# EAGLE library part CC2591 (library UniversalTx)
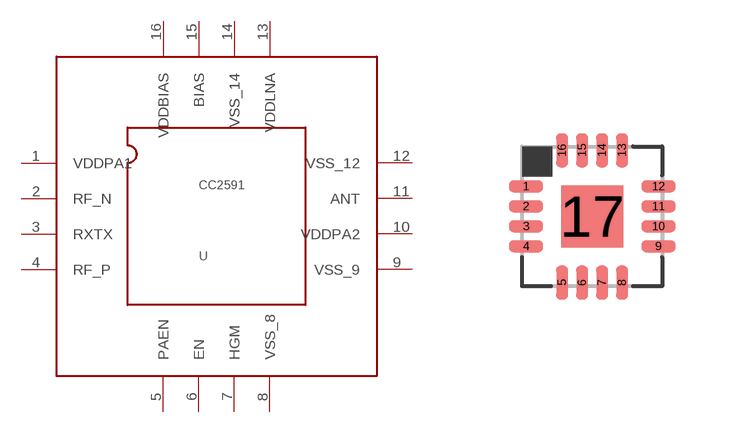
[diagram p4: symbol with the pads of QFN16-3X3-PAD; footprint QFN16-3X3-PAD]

Designator prefix -

## CC2591  [QFN16-3X3-PAD]
1  VDDPA1
2  RF_N
3  RXTX
4  RF_P
5  PAEN
6  EN
7  HGM
8  VSS_8
9  VSS_9
10  VDDPA2
11  ANT
12  VSS_12
13  VDDLNA
14  VSS_14
15  BIAS
16  VDDBIAS

## Footprint QFN16-3X3-PAD (pad centres in mm)
RTE (S-PQFP-N16) 3x3 mm Source: www.ti.com .. tpa6132a2 direct path stereo $.65.pdf
smd 0.85 x 0.3: 1 -1.655,0.75; 2 -1.655,0.25; 3 -1.655,-0.25; 4 -1.655,-0.75; 9 1.655,-0.75; 10 1.655,-0.25; 11 1.655,0.25; 12 1.655,0.75
smd 0.3 x 0.85: 5 -0.75,-1.655; 6 -0.25,-1.655; 7 0.25,-1.655; 8 0.75,-1.655; 13 0.75,1.655; 14 0.25,1.655; 15 -0.25,1.655; 16 -0.75,1.655
smd 1.55 x 1.55: 17 0,0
